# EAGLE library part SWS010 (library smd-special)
SMD Dip Switch 10 pol.
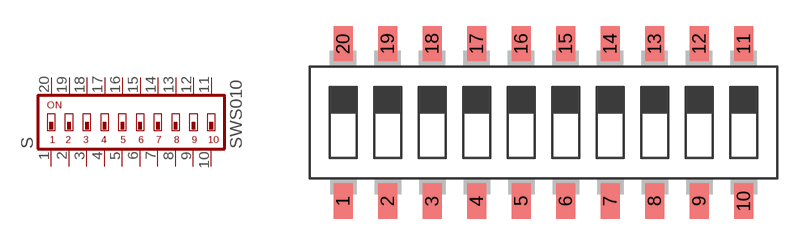
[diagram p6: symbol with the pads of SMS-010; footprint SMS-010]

Designator prefix S

## SWS010  [SMS-010]
1  1  pas
2  2  pas
3  3  pas
4  4  pas
5  5  pas
6  6  pas
7  7  pas
8  8  pas
9  9  pas
10  10  pas
11  11  pas
12  12  pas
13  13  pas
14  14  pas
15  15  pas
16  16  pas
17  17  pas
18  18  pas
19  19  pas
20  20  pas

## Footprint SMS-010 (pad centres in mm)
DIP SWITCH
smd 1.092 x 2.007: 1 -11.43,-4.496; 2 -8.89,-4.496; 3 -6.35,-4.496; 4 -3.81,-4.496; 5 -1.27,-4.496; 6 1.27,-4.496; 7 3.81,-4.496; 8 6.35,-4.496; 9 8.89,-4.496; 10 11.43,-4.496; 11 11.43,4.496; 12 8.89,4.496; 13 6.35,4.496; 14 3.81,4.496; 15 1.27,4.496; 16 -1.27,4.496; 17 -3.81,4.496; 18 -6.35,4.496; 19 -8.89,4.496; 20 -11.43,4.496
